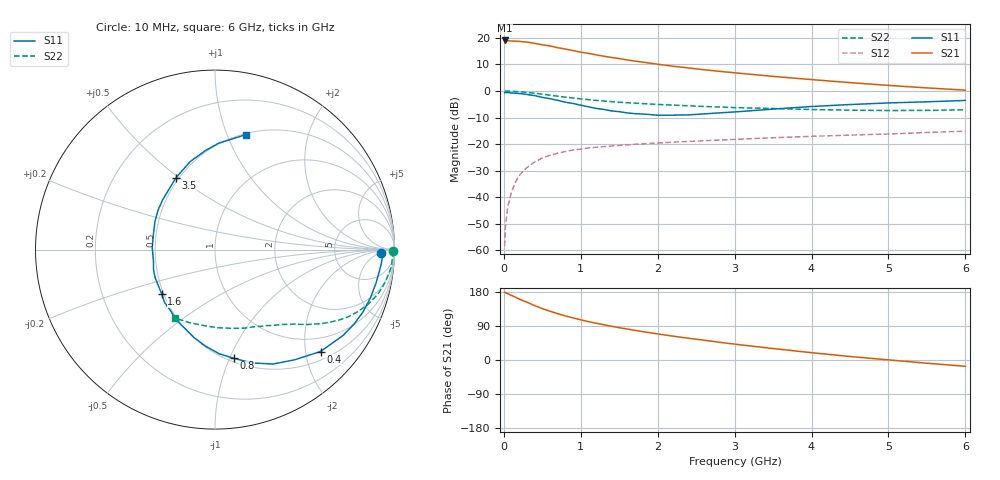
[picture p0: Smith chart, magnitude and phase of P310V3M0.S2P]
! SIEMENS Small Signal Semiconductors
! BFP181
! Si NPN RF Bipolar Junction Transistor in SOT143
! VCE = 10 V  IC = 3 mA
! Common Emitter S-Parameters:  March  1996
# GHz  S  MA  R  50
!  f  S11  S21  S12  S22
! GHz  MAG  ANG  MAG  ANG  MAG  ANG  MAG  ANG
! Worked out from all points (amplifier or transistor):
!   36 points, 10 MHz to 6 GHz, reference 50 ohm
!   highest |S21| = 19.0 dB at 10 MHz (marker M1)
!   |S21| within 3 dB of that: start of sweep to 753.8 MHz
!   unconditionally stable (mu >= 1): 2.288 GHz to end of sweep
!   at 250 MHz: K = 0.16, MSG = 24.4 dB, |S12| = -30.2 dB
!   at 1.4 GHz: K = 0.73, MSG = 16.7 dB, |S12| = -20.7 dB
!   at 6 GHz: K = 1.11, MAG = 5.7 dB, |S12| = -15.1 dB
!   S11 on the Smith chart (normalised r, x): 10 MHz: 24, -7; 400 MHz: 0.67, -2.31; 800 MHz: 0.53, -1.04; 1.6 GHz: 0.49, -0.28; 3.5 GHz: 0.48, +0.49; 6 GHz: 0.51, +1.17
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0.01  0.9272 -1.3  8.913 178.5  0.0012 68.7  0.9911 -0.5
0.02  0.9349 -2.4  8.906 178.1  0.0027 78.5  0.9919 -1.1
0.05  0.9287 -5.4  8.812 175.0  0.0066 89.2  0.9891 -2.7
0.1  0.9166 -11.6  8.704 170.4  0.0126 81.8  0.988 -5.4
0.2  0.895 -22.7  8.567 161.0  0.0253 77.3  0.9664 -10.6
0.25  0.8792 -28.1  8.423 156.4  0.0309 73.0  0.9533 -13.1
0.3  0.8591 -33.8  8.299 152.6  0.0362 70.0  0.9393 -15.5
0.4  0.8173 -44.0  7.867 143.6  0.0459 64.7  0.9056 -19.7
0.5  0.7577 -54.1  7.389 135.7  0.0547 59.6  0.8686 -23.4
0.6  0.7149 -63.1  7.02 128.7  0.0617 55.2  0.8311 -26.8
0.8  0.6146 -80.2  6.142 116.4  0.0724 48.0  0.7637 -31.8
0.9  0.5802 -87.8  5.749 111.1  0.0775 45.4  0.7362 -33.8
1.1  0.5032 -103.5  5.096 101.2  0.0846 41.0  0.6851 -37.2
1.3  0.4486 -118.6  4.501 93.0  0.0897 37.6  0.6458 -40.2
1.6  0.3868 -140.1  3.842 81.9  0.0966 34.1  0.6009 -43.7
1.9  0.3598 -162.2  3.339 71.9  0.1032 31.2  0.5676 -47.3
2.2  0.35 177.8  2.919 62.9  0.1085 29.3  0.5413 -51.0
2.8  0.3863 145.1  2.344 46.8  0.1191 25.9  0.4994 -58.9
3.5  0.4556 118.5  1.879 30.2  0.1317 22.4  0.467 -69.6
4.5  0.555 95.4  1.434 9.2  0.1474 16.9  0.4352 -88.6
5.5  0.6246 81.0  1.141 -8.5  0.1654 13.1  0.4311 -109.3
6  0.6623 75.1  1.034 -16.6  0.1749 10.3  0.4418 -120.1
